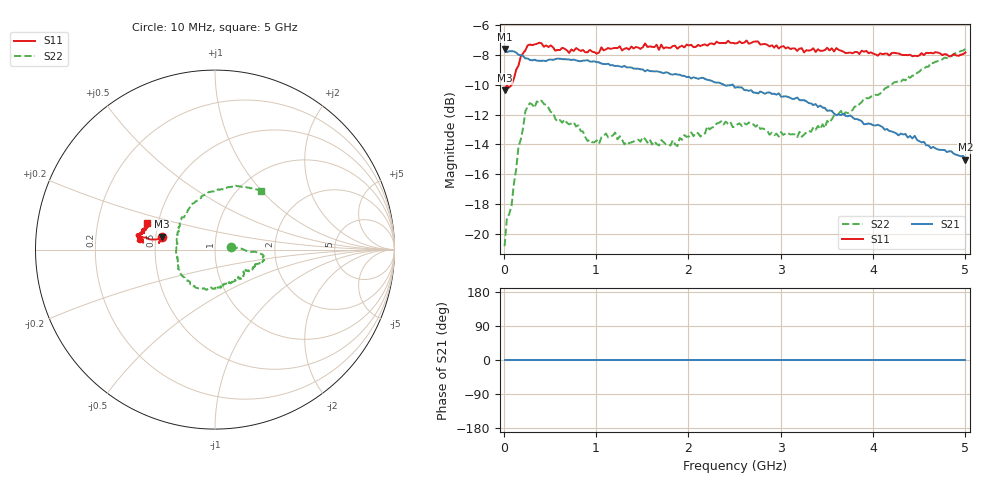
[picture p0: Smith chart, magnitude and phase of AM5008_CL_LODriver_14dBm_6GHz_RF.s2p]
!Keysight Technologies,N5245B,MY58422270,A.16.20.02
!Mixer S2P File: Scalar Mixer Measurement
!Calibration State: On
!Parameters: Stimulus Freq, S11, SC21, SC12, S22
# Hz  S  DB  R  50.0
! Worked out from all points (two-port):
!   201 points, 10 MHz to 5 GHz, reference 50 ohm
!   highest |S21| = -7.61 dB at 10 MHz (marker M1); lowest = -15.0 dB at 5 GHz (marker M2)
!   |S21| within 3 dB of the highest: start of sweep to 2.829 GHz; 2.83 GHz to 2.903 GHz (73.16 MHz wide, 2.55 % of centre)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
!   lowest |S11| = -10.4 dB at 10 MHz (marker M3), VSWR 1.87, Z = 27 + j4.31 ohm
!   |S11| at or under -10 dB: start of sweep to 86.12 MHz
!   |S22| runs from -20.8 to -7.6 dB; largest |S21 - S12| = 0.42
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1e7  -10.38 166.2  -7.61 0.0  -200.00 90.0  -20.82 9.7
3.495e7  -10.05 173.3  -7.82 0.0  -200.00 90.0  -18.94 2.9
8.485e7  -10.02 169.2  -7.75 0.0  -200.00 90.0  -18.12 4.9
1.597e8  -8.72 171.1  -7.99 0.0  -200.00 90.0  -14.19 -4.6
2.595e8  -7.37 169.9  -8.25 0.0  -200.00 90.0  -11.46 -6.1
4.092e8  -7.22 170.8  -8.40 0.0  -200.00 90.0  -11.07 -11.9
5.8385e8  -7.67 172.0  -8.25 0.0  -200.00 90.0  -12.47 -20.6
8.583e8  -7.68 173.4  -8.38 0.0  -200.00 90.0  -13.14 -31.7
1.03295e9  -7.84 173.2  -8.50 0.0  -200.00 90.0  -13.96 -38.6
1.2076e9  -7.54 173.4  -8.74 0.0  -200.00 90.0  -13.21 -48.1
1.3074e9  -7.59 173.9  -8.74 0.0  -200.00 90.0  -14.00 -49.5
1.68165e9  -7.67 172.8  -9.13 0.0  -200.00 90.0  -14.07 -67.3
1.88125e9  -7.59 172.9  -9.32 0.0  -200.00 90.0  -14.12 -78.1
2.2056e9  -7.39 171.2  -9.68 0.0  -200.00 90.0  -12.79 -101.8
2.505e9  -7.23 170.3  -10.21 0.0  -200.00 90.0  -12.80 -131.6
2.7545e9  -7.10 168.9  -10.59 0.0  -200.00 90.0  -12.67 -152.7
2.97905e9  -7.58 168.2  -10.58 0.0  -200.00 90.0  -13.47 -168.0
3.3533e9  -7.55 165.8  -11.37 0.0  -200.00 90.0  -12.86 159.2
3.6527e9  -7.72 164.4  -12.04 0.0  -200.00 90.0  -11.76 135.9
4.17665e9  -8.04 161.9  -13.10 0.0  -200.00 90.0  -10.10 99.4
4.62575e9  -7.85 159.8  -14.26 0.0  -200.00 90.0  -8.53 72.2
5e9  -7.85 158.1  -15.02 0.0  -200.00 90.0  -7.60 52.0
